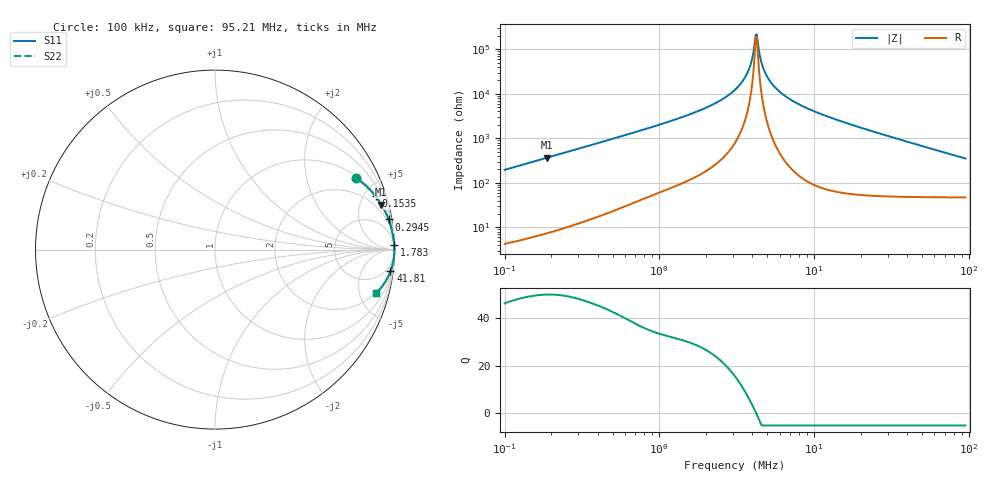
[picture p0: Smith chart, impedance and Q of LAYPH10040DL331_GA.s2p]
! LAYPH10040DL331_GA  S-PARAMETER MODEL  ( General Type )
! Model Generated by TAIYO YUDEN Corporation (http://www.ty-top.com)
! Version 1.0
! TAIYO YUDEN Control No. 180920NI43SB-FBB
! Copyright(c) 2018 TAIYO YUDEN CO.,LTD. All Rights Reserved.
! Product Description (link to TY-COMPAS)
! https://ds.yuden.co.jp/TYCOMPAS/or/detail?pn=LAYPH10040DL331MGA&u=M
! Products Name : Inductors
! Characteristics :
!  Inductance : 330 uH , SRF(min) : -Hz , DC Resistance(max) : 1.152 Ohm
!  Rated Current : Saturation :0.61 A , Temp Rise : 0.29 A (25 degC)
!  Case Size : 10.1 x 10.0 / 0.398 x 0.394 [mm/inch] , Thickness : 4 / 0.157 [mm/inch]
!  (Conditions: Temperature = 25 degC , DC Bias Current/Voltage = 0A / 0V)
! External Node Assignments :
!  1  o---GGG---o  2
! GND o---------o GND
! Frequency Range : 0.1MHz  -  95.211795MHz  [ 402 STEP ]
# MHz S RI R 50
! Freq[MHz].  S11 Real  S11 Imag  S21 Real  S21 Imag  S12 Real  S12 Imag  S22 Real  S22 Imag
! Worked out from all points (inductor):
!   401 points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, 100 kHz to 95.21 MHz, reference 50 ohm
!   read as one part in series: L = 310 uH near 103.5 kHz
!   highest Q = 49.6 at 188.6 kHz (marker M1), where L = 310 uH
!   self-resonance near 4.201 MHz
!   S11 on the Smith chart (normalised r, x): 100 kHz: 1.09, +3.91; 153.5 kHz: 1.12, +5.99; 294.5 kHz: 1, +11; 1.783 MHz: 4, +82; 41.81 MHz: 2, -16; 95.21 MHz: 1.94, -6.98
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0.1  0.7878 0.3981  0.2122 -0.3981  0.2122 -0.3981  0.7878 0.3981
0.153521  0.8948 0.2968  0.1052 -0.2968  0.1052 -0.2968  0.8948 0.2968
0.188594  0.9267 0.2508  0.0733 -0.2508  0.0733 -0.2508  0.9267 0.2508
0.29454  0.9672 0.1681  0.0328 -0.1681  0.0328 -0.1681  0.9672 0.1681
0.31545  0.971 0.1576  0.029 -0.1576  0.029 -0.1576  0.971 0.1576
0.995088  0.996 0.0496  0.00396 -0.0496  0.00396 -0.0496  0.996 0.0496
1.782584  0.9985 0.0244  0.00147 -0.0244  0.00147 -0.0244  0.9985 0.0244
2.469096  0.9992 0.0142  0.000842 -0.0142  0.000842 -0.0142  0.9992 0.0142
3.085641  0.9994 0.00813  0.000592 -0.00813  0.000592 -0.00813  0.9994 0.00813
3.419997  0.9995 0.00545  0.000513 -0.00545  0.000513 -0.00545  0.9995 0.00545
3.726142  0.9995 0.00326  0.000464 -0.00326  0.000464 -0.00326  0.9995 0.00326
3.922831  0.9996 0.00195  0.000441 -0.00195  0.000441 -0.00195  0.9996 0.00195
4.129902  0.9996 0.000653  0.000423 -0.000653  0.000423 -0.000653  0.9996 0.000653
4.273987  0.9996 -0.000214  0.000414 0.000214  0.000414 0.000214  0.9996 -0.000214
4.347904  0.9996 -0.000648  0.00041 0.000648  0.00041 0.000648  0.9996 -0.000648
4.737111  0.9996 -0.00283  0.000401 0.00283  0.000401 0.00283  0.9996 -0.00283
5.341222  0.9996 -0.00592  0.000414 0.00592  0.000414 0.00592  0.9996 -0.00592
6.790391  0.9995 -0.0124  0.000542 0.0124  0.000542 0.0124  0.9995 -0.0124
9.733658  0.9989 -0.0237  0.00109 0.0237  0.00109 0.0237  0.9989 -0.0237
30.70484  0.9879 -0.0892  0.0121 0.0892  0.0121 0.0892  0.9879 -0.0892
41.80689  0.9777 -0.1206  0.0223 0.1206  0.0223 0.1206  0.9777 -0.1206
95.21179  0.8974 -0.2433  0.1026 0.2433  0.1026 0.2433  0.8974 -0.2433
